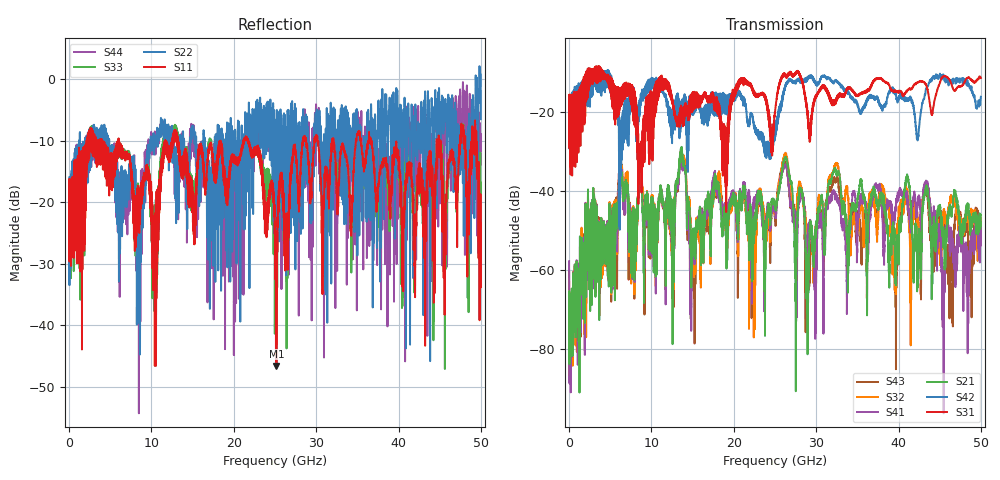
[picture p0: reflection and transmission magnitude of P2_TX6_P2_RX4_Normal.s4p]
!Keysight Technologies,N5225B,MY57041031,A.13.20.10
!Date: Friday, May 31, 2019 11:32:57
!Correction: S11(Full 4 Port(1,2,3,4))
!S12(Full 4 Port(1,2,3,4))
!S13(Full 4 Port(1,2,3,4))
!S14(Full 4 Port(1,2,3,4))
!S21(Full 4 Port(1,2,3,4))
!S22(Full 4 Port(1,2,3,4))
!S23(Full 4 Port(1,2,3,4))
!S24(Full 4 Port(1,2,3,4))
!S31(Full 4 Port(1,2,3,4))
!S32(Full 4 Port(1,2,3,4))
!S33(Full 4 Port(1,2,3,4))
!S34(Full 4 Port(1,2,3,4))
!S41(Full 4 Port(1,2,3,4))
!S42(Full 4 Port(1,2,3,4))
!S43(Full 4 Port(1,2,3,4))
!S44(Full 4 Port(1,2,3,4))
!S4P File: Measurements: <S11,S12,S13,S14>,
!<S21,S22,S23,S24>,
!<S31,S32,S33,S34>,
!<S41,S42,S43,S44>:
# Hz S  dB  R 50.0
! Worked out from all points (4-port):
!   5000 points, 10 MHz to 50 GHz, reference 50 ohm
!   strongest paths, dB at 10 MHz, 12.51 GHz, 25.01 GHz, 37.51 GHz, 50 GHz:
!     S31: -19.3, -16.8, -20.0, -11.6, -11.4
!     S42: -19.6, -27.9, -23.8, -16.9, -16.2
!     S21: -66.8, -47.4, -43.2, -44.3, -46.0
!     S41: -57.7, -48.9, -43.8, -40.0, -53.8
!     S32: -64.8, -47.9, -44.0, -47.6, -46.9
!     S43: -60.4, -49.5, -45.9, -43.9, -51.6
!   lowest |S11| = -46.6 dB at 25.18 GHz (marker M1), VSWR 1.01, Z = 50 - j0.469 ohm
!   |S11| at or under -10 dB: 13.21 GHz to 21.18 GHz (7.965 GHz wide, 46.3 % of centre); 21.74 GHz to 28.38 GHz (6.639 GHz wide, 26.5 % of centre); 36.67 GHz to 44.63 GHz (7.963 GHz wide, 19.6 % of centre)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
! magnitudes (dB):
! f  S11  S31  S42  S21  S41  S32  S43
! 10 MHz  -19.4  -19.3  -19.6  -66.8  -57.7  -64.8  -60.4
! 6.27 GHz  -10.6  -14.1  -25.7  -38.0  -36.6  -35.3  -34.6
! 7.73 GHz  -19.4  -20.1  -14.7  -50.9  -50.3  -51.2  -51.1
! 13.78 GHz  -16.2  -20.1  -17.3  -32.9  -34.8  -32.2  -33.8
! 14.95 GHz  -21.1  -15.6  -17.7  -52.3  -53.3  -51.6  -52.7
! 25.18 GHz  -46.6  -16.9  -23.8  -43.7  -44.9  -43.7  -43.4
! 50 GHz  -23.5  -11.4  -16.2  -46.0  -53.8  -46.9  -51.6
